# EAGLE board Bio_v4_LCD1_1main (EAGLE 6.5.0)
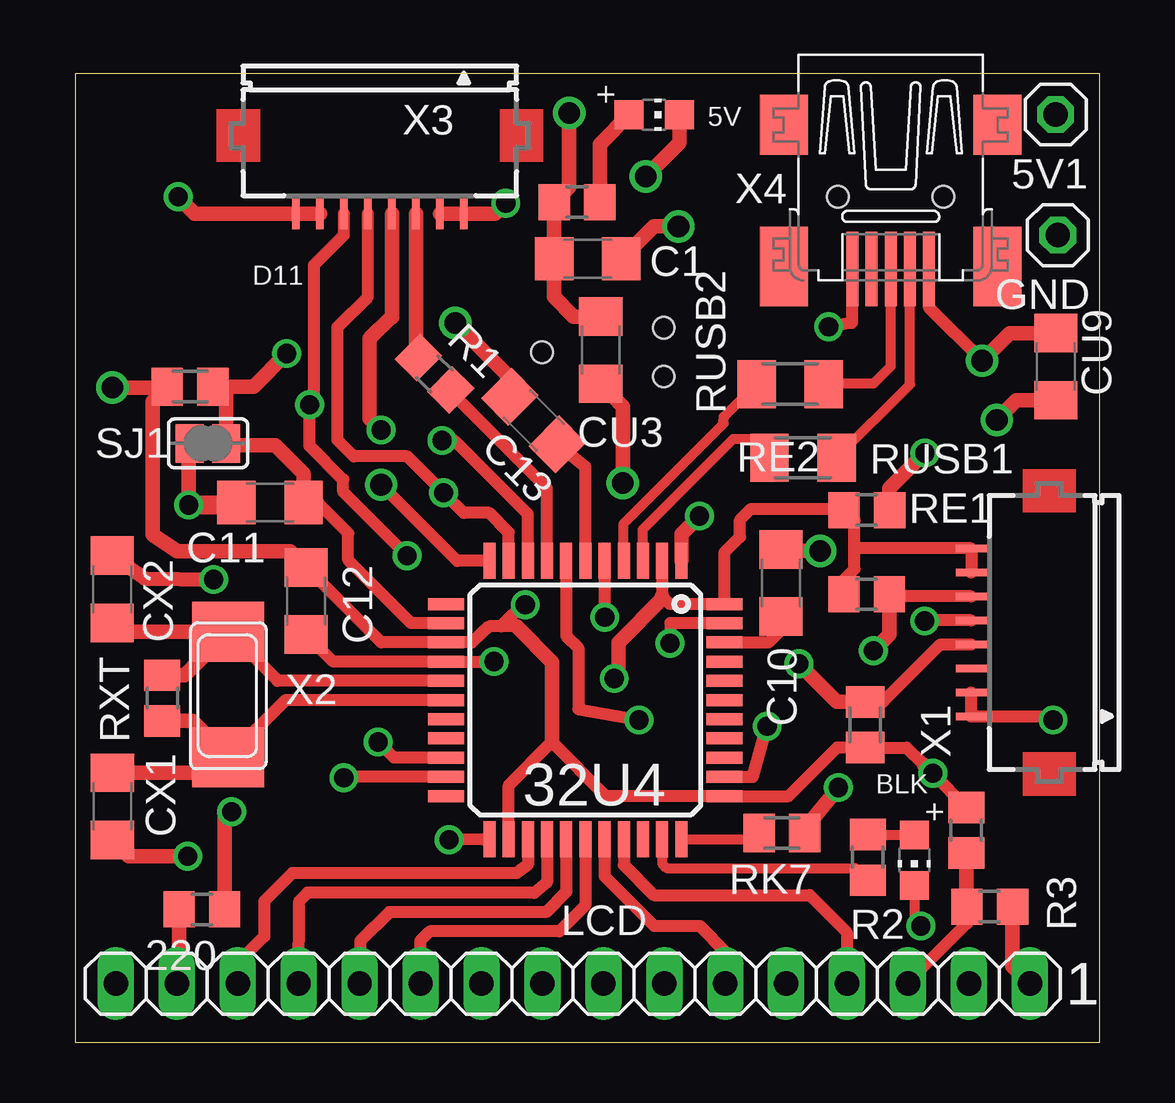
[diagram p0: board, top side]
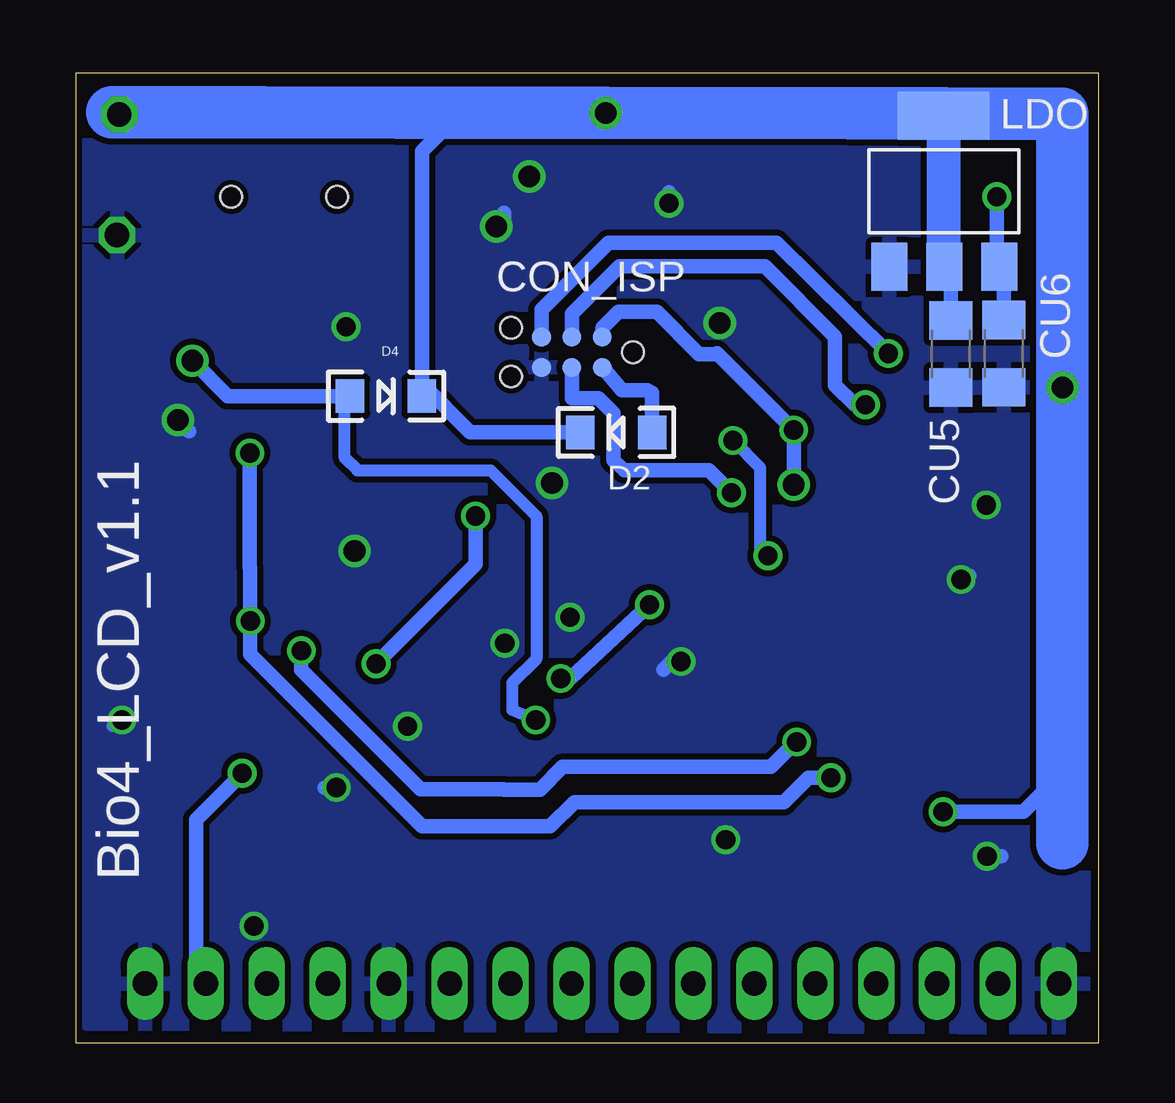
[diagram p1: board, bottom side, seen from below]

Size 42.66 x 40.41 mm. Coordinates in mm from the lower left corner, seen from the top.
Outline: 42.66,0 0,0 0,40.41 42.66,40.41 42.66,19.56 42.66,19.52 42.66,0
Copper layers (1*2*15*16): Top 0.035mm / dielectric 0.2mm / layer 2 0.0175mm / dielectric 1.1mm / layer 15 0.0175mm / dielectric 0.2mm / Bottom 0.035mm
Design rules "SeeedStudio_DRU_no_angle_20130527": minimum track width 6mil, minimum drill 12mil, track to track 6mil, track to pad 6mil, pad to pad 6mil, via to via 6mil, smd to smd 0mil, copper to edge 10mil, drill to drill 10mil, minimum pad ring 6mil, minimum via ring 6mil, stop-mask expansion 2mil, vias tented up to drill 25mil, thermal gap 10mil
Net classes: 0 default: width 0.203 mm, clearance 0.25 mm; 1 power: width 0.203 mm, drill 0.305 mm, clearance 0.25 mm; 2 VIN: width 0.457 mm, clearance 0.25 mm; 3 fine: width 0.254 mm, clearance 0.25 mm; 4 aref: width 0.356 mm, clearance 0.25 mm
vRestrict: area 8.7,33.5 to 16.8,37.3

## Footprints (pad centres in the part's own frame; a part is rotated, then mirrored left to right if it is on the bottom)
1X01 = drill 1.016 octagon: 1 0,0
TQFP44 = smd 1.5 x 0.5: 1 -5.8,4; 2 -5.8,3.2; 3 -5.8,2.4; 4 -5.8,1.6; 5 -5.8,0.8; 6 -5.8,0; 7 -5.8,-0.8; 8 -5.8,-1.6; 9 -5.8,-2.4; 10 -5.8,-3.2; 11 -5.8,-4; 23 5.8,-4; 24 5.8,-3.2; 25 5.8,-2.4; 26 5.8,-1.6; 27 5.8,-0.8; 28 5.8,0; 29 5.8,0.8; 30 5.8,1.6; 31 5.8,2.4; 32 5.8,3.2; 33 5.8,4 | smd 0.5 x 1.5: 12 -4,-5.8; 13 -3.2,-5.8; 14 -2.4,-5.8; 15 -1.6,-5.8; 16 -0.8,-5.8; 17 0,-5.8; 18 0.8,-5.8; 19 1.6,-5.8; 20 2.4,-5.8; 21 3.2,-5.8; 22 4,-5.8; 34 4,5.8; 35 3.2,5.8; 36 2.4,5.8; 37 1.6,5.8; 38 0.8,5.8; 39 0,5.8; 40 -0.8,5.8; 41 -1.6,5.8; 42 -2.4,5.8; 43 -3.2,5.8; 44 -4,5.8
R0805 = smd 1.3 x 1.5: 1 -0.95,0; 2 0.95,0
CHIP-LED0805 = smd 1.2 x 1.2: A 0,-1.05; C 0,1.05
C1206 = smd 1.6 x 1.8: 1 -1.4,0; 2 1.4,0
TC2030-MCP-NL = smd 0.787 x 0.787: 5V 1.27,0.635; GND 3.81,0.635; MISO 1.27,-0.635; MOSI 2.54,0.635; RESET 3.81,-0.635; SCK 2.54,-0.635 | hole 0.889: 0,0; 5.08,-1.016; 5.08,1.016
LED-1206 = smd 1.2 x 1.4: A -1.5,0; C 1.5,0
1X16 = drill 1.016 long: 1 -19.05,0; 2 -16.51,0; 3 -13.97,0; 4 -11.43,0; 5 -8.89,0; 6 -6.35,0; 7 -3.81,0; 8 -1.27,0; 9 1.27,0; 10 3.81,0; 11 6.35,0; 12 8.89,0; 13 11.43,0; 14 13.97,0; 15 16.51,0; 16 19.05,0
SOT223 = smd 1.499 x 2.007: 1 -2.261,-3.15; 2 0.025,-3.15; 3 2.311,-3.15 | smd 3.81 x 2.007: 4 0,3.15
M0805 = smd 1.3 x 1.6: 1 -0.95,0; 2 0.95,0
M1206 = smd 1.6 x 2: 1 -1.4,0; 2 1.4,0
SJ = smd 1.168 x 1.6: 1 -0.762,0; 2 0.762,0
FH12-08S-1SH = smd 0.3 x 1.3: 1 -3.5,3.25; 2 -2.5,3.25; 3 -1.5,3.25; 4 -0.5,3.25; 5 0.5,3.25; 6 1.5,3.25; 7 2.5,3.25; 8 3.5,3.25
NX6035 = smd 2.5 x 3: P$1 2.665,0; P$2 -2.565,0
32005-201 = smd 3.1 x 0.5: 1 3,1.6; 2 3,0.8; 3 3,0; 4 3,-0.8; 5 3,-1.6 | smd 2.5 x 2: M1 -3,-4.45; M2 -3,4.45 | smd 3.3 x 2: M3 2.9,4.45; M4 2.9,-4.45 | hole 0.9: 0,2.2; 0,-2.2

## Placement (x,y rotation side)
5V1  [1X01]  40.84,38.68 180 top
32U4  32U4  [TQFP44]  21.24,14.29 270 top
220  220  [R0805]  5.25,5.56 180 top
BKLD  RED  [CHIP-LED0805]  34.95,7.61 180 top
C1  100nF  [C1206]  21.34,32.67 0 top
C10  100nF  [C1206]  29.39,19.16 90 top
C11  100nF  [C1206]  8.1,22.52 180 top
C12  100nF  [C1206]  9.6,18.41 90 top
C13  100nF  [C1206]  19.08,25.93 315 top
CON_ISP  SPI  [TC2030-MCP-NL]  19.43,28.78 180 bottom
CU3  10uF  [C1206]  21.88,28.87 270 top
CU5  10uF  [C1206]  6.17,28.71 270 bottom
CU6  10uF  [C1206]  3.97,28.72 270 bottom
CU9  10uF  [C1206]  40.84,28.18 90 top
CX1  22pF  [C1206]  1.53,9.86 90 top
CX2  22pF  [C1206]  1.52,18.9 270 top
D2  1N581D1206  [LED-1206]  20.12,25.44 180 bottom
D4  1N581D1206  [LED-1206]  29.73,26.95 0 bottom
GND  [1X01]  40.93,33.66 180 top
LCD  [1X16]  20.72,2.47 180 top
LDO  NCP1117LPST50T3G  [SOT223]  6.47,35.48 0 bottom
LDPW5  RED  [CHIP-LED0805]  24.11,38.67 270 top
R1  1k  [R0805]  14.95,27.88 315 top
R2  1k  [R0805]  33.01,7.73 90 top
R3  1k  [R0805]  38.09,5.68 0 top
R13  1k  [R0805]  20.89,35.04 0 top
RE1  5k  [R0805]  32.97,22.2 0 top
RE2  5k  [R0805]  32.96,18.69 0 top
RK1  10k  [R0805]  37.12,8.86 270 top
RK2  10k  [M0805]  32.9,13.25 270 top
RK6  10k  [M0805]  4.76,27.34 180 top
RK7  10k  [M0805]  29.43,8.74 180 top
RUSB1  22  [M1206]  30.31,24.38 0 top
RUSB2  22  [M1206]  29.77,27.45 0 top
RXT  1M  [R0805]  3.6,14.37 270 top
SJ1  [SJ]  5.51,24.98 0 top
X1  FH12-08S-1SH  [FH12-08S-1SH]  40.57,17.1 90 top
X2  16MHz  [NX6035]  6.36,14.46 90 top
X3  FH12-08S-1SH  [FH12-08S-1SH]  12.67,37.81 180 top
X4  MINI-USB  [32005-201]  33.97,35.25 270 top

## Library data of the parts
5V1 GND = Headerlibrary
32U4 BKLD LDPW5 = adafruit
220 C1 C10-C13 CU3 CU5 CU6 CU9 CX1 CX2 R1-R3 RE1 RE2 RK1 RXT = rcl
CON_ISP D2 D4 LCD LDO X2 = lpatiny
R13 RK2 RK6 RK7 RUSB1 RUSB2 = resistor
SJ1 = jumper
X1 X3 = con-hirose; OC_FARNELL: unknown; OC_NEWARK: unknown
X4 = con-cypressindustries; OC_FARNELL: unknown; OC_NEWARK: unknown

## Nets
+5V/1 [fine]: 5V1.1 32U4.2 32U4.14 32U4.24 32U4.34 32U4.44 220.1 C1.1 C12.2 CU3.1 CU5.1 D2.C D4.C LCD.2 LDO.2 LDO.4 R13.1 RE1.1 RE2.1 RK1.1 RK2.2 RK6.2 X1.7 X1.8
+12V [power]: CU6.1 LDO.3 X3.7 X3.8
A0: 32U4.36
A1: 32U4.37
A2: 32U4.38
A3: 32U4.39
A4: 32U4.40
A5: 32U4.41
A6: 32U4.25 LCD.14
AREF: 32U4.42 C10.1
CS_32U4: R1.1 X3.3
D5*: 32U4.31
D6*: 32U4.27 LCD.12
D7*: 32U4.1 RK2.1 X1.4
D8*: 32U4.28 LCD.11
D9*: 32U4.29 LCD.6
D10*: 32U4.30 LCD.4
D11*: 32U4.12
D12*: 32U4.26 LCD.13
D13*: 32U4.32 R2.1
GND [power]: 32U4.5 32U4.15 32U4.23 32U4.35 32U4.43 BKLD.C C1.2 C10.2 C11.2 C12.1 C13.1 CON_ISP.GND CU3.2 CU5.2 CU6.2 CU9.1 CX1.1 CX2.1 GND.1 LCD.1 LCD.5 LCD.16 LDO.1 LDPW5.C R3.2 RK7.1 SJ1.1 X1.1 X1.2 X3.1 X3.2 X4.5
HWB: 32U4.33 RK7.2
ISP+5V: CON_ISP.5V D2.A
MISO: 32U4.11 CON_ISP.MISO X3.4
MOSI: 32U4.10 CON_ISP.MOSI X3.5
N$1: 32U4.6 C13.2
N$2: LCD.3 R3.1 RK1.2
N$3: BKLD.A R2.2
N$11: 220.2 LCD.15
N$12: LDPW5.A R13.2
N$42: 32U4.17 CX1.2 RXT.2 X2.P$2
RESET: 32U4.13 C11.1 CON_ISP.RESET RK6.1 SJ1.2
RX: 32U4.20 RE2.2 X1.6
RXLED: 32U4.8 R1.2
SCK: 32U4.9 CON_ISP.SCK X3.6
SCL: 32U4.18
SDA: 32U4.19
TX: 32U4.21 RE1.2 X1.5
TXLED: 32U4.22
USB_N: 32U4.3 RUSB1.1
USB_P: 32U4.4 RUSB2.1
USBC_N: RUSB1.2 X4.2
USBC_P: RUSB2.2 X4.3
VUSB: 32U4.7 CU9.2 D4.A X4.1
XTAL1: 32U4.16 CX2.2 RXT.1 X2.P$1

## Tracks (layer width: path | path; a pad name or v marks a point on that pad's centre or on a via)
+5V/1  (via drill 0.8, 0.8 pad 0.81, 0.9, 0.9 pad 0.61)
  Top 0.5: 32U4.24 18.04,10.72 19.85,12.54 22.11,10.29 32U4.34 29.71,10.29 31.73,12.3 RK2.2 34.62,12.3 35.35,11.6 | 18.36,17.35 17.73,17.35 | 17.73,17.35 17.23,17.35 16.51,16.69 15.45,16.69 32U4.14 12.73,16.69 C12.2 | 32U4.2 24.44,18.6 24.76,18.29 32U4.44 27.04,20.44 27.68,21.09 27.68,21.79 28.14,22.25 31.98,22.25 RE1.1 32.45,21.77 32.45,20.58 | 18.74,18.36 17.73,17.35 | RK1.1 v35.72,11.23 | RE2.1 32.01,19.29 32.45,19.74 32.45,20.58 | 32.45,20.58 32.47,20.6 X1.8 X1.7
  Top 0.61: 19.85,12.54 19.85,15.86 18.36,17.35 | C12.2 8.93,20.48 4.23,20.48 3.21,21.18 3.21,26.74 3.78,27.3 | 24.44,18.6 24.44,18.5 22.62,16.68 22.62,15.37 v22.44,15.18 | v18.74,18.26 18.74,18.36 | RK6.2 3.78,27.3 | 3.78,27.3 v1.52,27.3 | v20.56,38.75 20.56,35.66 R13.1 C1.1 19.93,31.09 20.75,30.27 CU3.1 | 220.1 6.2,9.34 v6.49,9.63 | 36.89,10.04 RK1.1 | v35.72,11.23 35.35,11.6
  Bottom 0.254: 5V1.1 41.42,38.88 41.13,38.77
  Bottom 0.61: v22.44,15.18 22.04,15.18 v18.74,18.26 | 1.52,38 1.52,38.35 1.88,38.71 | v20.56,38.75 v20.57,38.75 21.06,38.75 | v6.49,9.63 3.15,9.63 1.52,11.26 | D4.C 28.23,27.46 | 28.23,27.46 28.23,37.14 26.61,38.76 | D2.C 26.21,25.44 28.23,27.46 | 9.86,38.73 10.37,38.73 | CU5.1 6.17,32.06 LDO.2 | LCD.2 37.63,2.87 37.63,9.29 36.07,10.85 v35.72,11.23
  Bottom 1.422: LDO.2 6.47,32.33 LDO.4
  Bottom 2.184: 1.52,8.31 1.52,8.8 1.52,11.26 v1.52,27.3 1.52,38 1.52,38.71 1.88,38.71 6.47,38.71 LDO.4 6.47,38.73 9.86,38.73 10.37,38.73 v20.56,38.75 21.06,38.75 25.49,38.76 26.61,38.76 29.21,38.76 34.88,38.77 41.13,38.77
+12V  (via drill 0.8)
  Top 0.61: X3.7 X3.8 4.96,34.55 v4.26,35.25
  Bottom 0.61: v4.26,35.25 4.26,32.44 LDO.3 3.97,32.15 CU6.1
A6
  Top 0.5: 32U4.25 18.84,7.42 18.37,7.07 9.02,7.07 7.85,5.91 7.85,4.44 6.93,3.52 6.93,2.32 LCD.14
AREF
  Top 0.5: 32U4.42 28.86,16.69 28.87,16.67 29.32,17.13 C10.1
CS_32U4
  Top 0.61: X3.3 14.17,28.65 R1.1
D6*
  Top 0.5: 32U4.27 20.44,6.29 19.6,5.45 13.07,5.45 11.86,4.24 11.86,2.18 LCD.12
D7*  (via drill 0.8)
  Top 0.5: RK2.1 33.65,14.2 36.05,16.6 X1.4
  Top 0.61: 32U4.1 25.24,21.2 v25.99,21.95 | v30.14,15.79 31.73,14.2 RK2.1
  Bottom 0.61: v25.99,21.95 25.99,19.94 v30.14,15.79
D8*
  Top 0.5: 32U4.28 21.24,5.73 20.16,4.65 14.75,4.65 14.35,4.25 14.35,2.49
  Top 0.61: 14.35,2.49 LCD.11
D9*
  Top 0.5: 32U4.29 22.04,6.94 24.1,4.88 26,4.88 27.09,3.79 27.09,2.49
  Top 0.61: 27.09,2.49 LCD.6
D10*
  Top 0.5: 32U4.30 22.84,7.4 24.08,6.16 30.59,6.16 32.14,4.61 32.14,2.48
  Top 0.61: 32.14,2.48 LCD.4
D12*
  Top 0.5: 32U4.26 19.64,6.68 19.12,6.25 11.68,6.26 9.66,6.26 9.31,5.91 LCD.13
D13*
  Top 0.406: 32U4.32 24.44,7.49 24.62,7.28 32.48,7.28 R2.1
GND  (via drill 0.8, 0.8 pad 0.81, 0.9, 0.9 pad 0.81)
  Top 0.406: BKLD.C 34.95,5.14 v35.22,4.87
  Top 0.5: v17.43,15.89 17.35,15.87 32U4.15 10.73,15.89 C12.1 | 32U4.5 22.04,18.36 v22.05,17.74 | 32U4.23 16.97,8.48 v15.56,8.47 | 32U4.43 24.78,17.49 v24.77,16.65 | v31.38,29.84 32.35,30 32.37,30.02 X4.5 | 32U4.35 28.22,11.09 v28.82,13.19 | v40.73,13.45 40.59,13.6 X1.1 X1.2
  Top 0.61: CX2.1 2.89,19.34 v5.75,19.31 | v4.66,7.78 2.21,7.78 CX1.1 | C10.2 29.45,20.5 v31.03,20.5 | SJ1.1 4.7,24.93 v4.7,22.41 | LDPW5.C 25.16,37.5 v23.75,36.09 | C1.2 24.09,34.02 v25.12,34.02 | CU3.2 22.8,26.51 v22.8,23.32 | CU9.1 39.21,26.78 v38.39,25.96 | RK7.1 30.56,9.13 v31.79,10.64 | LCD.1 39.04,3.2 R3.2 | C13.1 18.09,27.72 v15.82,30 | X3.2 X3.1 17.48,34.55 v17.92,34.99
  Top 0.813: C11.2 6.54,22.42 v4.7,22.41
  Bottom 0.406: v35.22,4.87 35.22,4.95 35.34,5.07
  Bottom 0.5: v17.43,15.89 17.82,15.88 | v40.73,13.45 40.87,13.45 41.12,13.2
  Bottom 0.61: 17.82,15.88 18.16,15.55 | v4.66,7.78 4.07,7.78 | v5.75,19.31 5.54,19.32 5.41,19.46 | v23.75,36.09 23.89,36.09 23.91,36.11 | v25.12,34.02 24.81,34.34 24.81,34.59 | v22.8,23.32 23.07,23.53 22.97,23.29 | v38.39,25.96 | v38.39,25.96 37.92,25.48 | v31.79,10.64 32.27,10.64 | v17.92,34.99 17.92,35.44
  pour Bottom: 0.44,39.86 0.4,39.89 0.67,0.63 42.17,0.79 42.17,20.07 42.36,20.69 42.36,40.6 1.7,40.25 0.68,40.13
HWB
  Top 0.406: 32U4.33 28.23,8.49 RK7.2
ISP+5V
  Bottom 0.61: CON_ISP.5V 19.87,27.19 18.83,27.19 18.64,27.08 18.64,25.46 D2.A
MISO  (via drill 0.8, 0.9 pad 0.61)
  Top 0.5: 32U4.11 15.89,20.09 v12.72,23.25
  Top 0.61: X3.4 13.19,34.54 13.19,30.24 13.14,30.24 12.26,29.35 12.26,26.01 v12.72,25.54
  Bottom 0.61: v12.72,23.25 v12.72,25.54 15.92,28.74 15.96,28.7 16.67,28.7 18.44,30.46 20.03,30.46 20.7,29.79 CON_ISP.MISO
MOSI  (via drill 0.8)
  Top 0.5: 32U4.10 18.04,21.27 17.23,22.08 16.17,22.08 v15.32,22.92 13.82,24.43 11.59,24.43 10.91,25.11 10.91,29.83 12.17,31.09 X3.5
  Bottom 0.61: CON_ISP.MOSI 21.97,26.86 20.87,26.86 20.25,26.24 20.25,24.28 20.16,24.19 19.78,23.85 16.25,23.85 v15.32,22.92
N$1
  Top 0.5: 32U4.6 21.24,24.01 C13.2
N$2
  Top 0.5: 34.69,2.53 37.14,4.98 R3.1
  Top 0.61: LCD.3 34.69,2.53 | R3.1 37.12,5.71 RK1.2
N$3
  Top 0.406: R2.2 34.93,8.68 BKLD.A
N$11
  Top 0.61: 220.2 4.3,2.23 LCD.15
N$12
  Top 0.61: R13.2 21.84,37.45 LDPW5.A
N$42
  Top 0.5: 32U4.17 8.75,14.29 X2.P$2
  Top 0.61: CX1.2 6.37,11.26 6.96,11.85 6.41,11.85 X2.P$2 4.84,13.42 RXT.2
RESET  (via drill 0.8 pad 0.81)
  Top 0.5: 32U4.13 13.98,17.49 11.35,20.11 11.35,21.23 10.05,22.53
  Top 0.61: 9.62,22.39 C11.1 | C11.1 9.49,23.72 8.31,24.9 6.35,24.9 SJ1.2 6.27,27.34 RK6.1 7.42,27.34 v8.78,28.73 | 10.05,22.53 9.51,22.53 C11.1
  Bottom 0.61: CON_ISP.RESET 23.24,30.55 20.45,33.34 13.44,33.34 v8.78,28.73
RX  (via drill 0.8)
  Top 0.5: 32U4.20 13.26,11.89 v12.6,12.54 | X1.6 34.01,18.6
  Top 0.61: v33.25,16.34 33.91,17 RE2.2 34.01,18.6
  Bottom 0.61: v12.6,12.54 12.64,12.54 13.68,11.5 22.35,11.5 23.29,10.56 24.79,10.56 24.81,10.58 28.29,10.58 33.25,15.54 v33.25,16.34
RXLED
  Top 0.5: 32U4.8 19.64,23.11 15.62,27.12
  Top 0.61: R1.2 15.62,27.12
SCK  (via drill 0.8)
  Top 0.5: 32U4.9 18.84,22.02 15.76,25.1 v15.26,25.1 | X3.6 11.17,33.66 9.92,32.41 9.92,26.77 v9.74,26.58 9.74,24.87 11.15,23.47 11.15,22.95 v13.8,20.3
  Bottom 0.5: v15.26,25.1 14.13,23.96 14.13,20.3 v13.8,20.3
  Bottom 0.61: CON_ISP.SCK 21.96,30.39 19.99,32.36 13.94,32.36 11.01,29.43 11.01,27.41 10.18,26.58 v9.74,26.58
SCL
  Top 0.5: 15.45,13.49 32U4.18
TX  (via drill 0.8)
  Top 0.5: 32U4.21 11.22,11.09 v11.17,11.04 | X1.5 35.4,17.6 v35.38,17.58
  Top 0.61: v35.39,24.58 33.92,23.11 RE1.2
  Bottom 0.61: v11.17,11.04 12.11,11.04 13.12,10.03 21.87,10.03 22.88,9.02 28.21,9.02 35.38,16.19 v35.38,17.58 35.38,19.8 35.39,19.82 v35.39,24.58
USB_N
  Top 0.406: 32U4.3 23.64,21.39 27.41,25.16 28.12,25.16 RUSB1.1
USB_P
  Top 0.406: RUSB2.1 27.01,26.09 27,25.83 27,25.8 22.84,21.64 32U4.4
USBC_N
  Top 0.406: X4.2 34.77,27.43 RUSB1.2
USBC_P
  Top 0.406: X4.3 33.97,28.19 33.25,27.47 31.19,27.47 RUSB2.2
VUSB  (via drill 0.8 pad 0.81, 0.9)
  Top 0.5: 32U4.7 20.44,16.97 20.94,16.46 20.94,13.91 v23.48,13.46 | v37.78,28.42 35.57,30.64 X4.1
  Top 0.61: CU9.2 38.94,29.58 v37.78,28.42
  Bottom 0.5: 23.47,13.38 v23.48,13.46 24.46,13.88 24.46,14.99 23.46,15.99 23.46,21.95 25.36,23.85 30.92,23.85 31.44,24.38 31.44,26.74
  Bottom 0.61: D4.A 36.31,26.95 v37.78,28.42 | D4.A 31.23,26.88 | 31.44,26.74 D4.A
XTAL1
  Top 0.5: 32U4.16 8.4,15.09 X2.P$1
  Top 0.61: CX2.2 1.9,17.13 X2.P$1 4.55,15.32 RXT.1

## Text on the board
tNames: 5V | D11 | BLK | 1
bNames: Bio4_LCD_v1.1
tValues: Screen / v0.1
203bmp: C:/Users/G/Pictures/logo_epfl.bmp

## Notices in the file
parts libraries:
lpatiny: ©2009 ROFA.cz - modified and updated by Robert Darlington ‹rdarlington@gmail.com›
